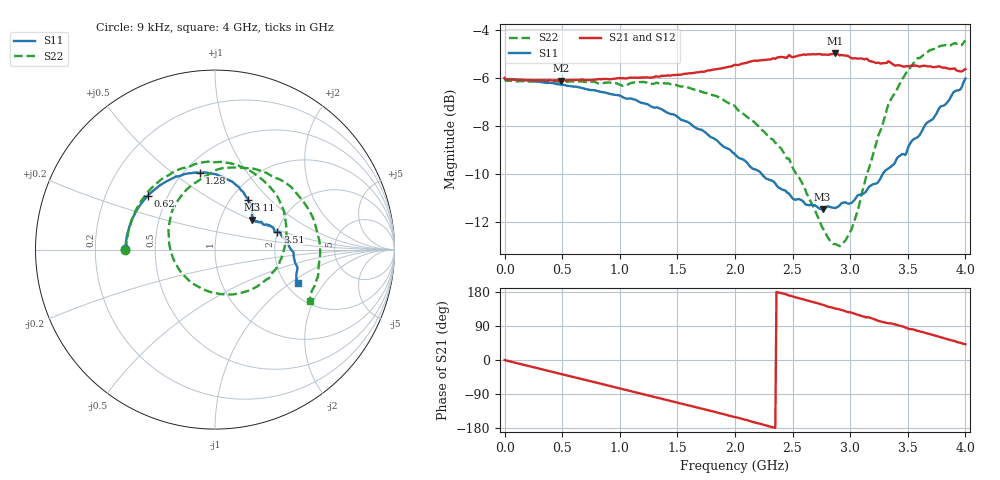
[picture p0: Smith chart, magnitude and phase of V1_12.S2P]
! ZVRE, 3.40
! symbol freq-unit parameter-type data-format keyword impedance-ohm
#  HZ  S  RI  R  50
! freq  reS11  imS11  reS21  imS21  reS12  imS12  reS22  imS22
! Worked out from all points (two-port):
!   401 points, 9 kHz to 4 GHz, reference 50 ohm
!   highest |S21| = -4.96 dB at 2.87 GHz (marker M1); lowest = -6.1 dB at 490 MHz (marker M2)
!   |S21| within 3 dB of the highest: start of sweep to end of sweep
!   lowest |S11| = -11.5 dB at 2.76 GHz (marker M3), VSWR 1.73, Z = 70.9 + j25.5 ohm
!   |S11| at or under -10 dB: 2.232 GHz to 3.283 GHz (1.051 GHz wide, 38.1 % of centre)
!   |S22| runs from -13.0 to -4.4 dB; largest |S21 - S12| = 0.02
!   S11 on the Smith chart (normalised r, x): 9 kHz: 0.33, +0.00; 620 MHz: 0.39, +0.30; 1.28 GHz: 0.59, +0.63; 2.11 GHz: 1.19, +0.75; 3.51 GHz: 2.00, +0.46; 4 GHz: 2.34, -1.15
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9000  -0.4999 0.000718  0.5014 0.000349  0.5019 -0.00206  -0.5 -0.000897
4.900079e8  -0.4173 0.2476  0.3952 -0.2977  0.3997 -0.2964  -0.407 0.2766
6.200076e8  -0.3754 0.3004  0.3407 -0.3608  0.3453 -0.3613  -0.3588 0.3379
6.700075e8  -0.3573 0.3171  0.3165 -0.3831  0.3216 -0.3821  -0.3364 0.3597
9.900068e8  -0.2215 0.4047  0.1363 -0.4818  0.1393 -0.4839  -0.1703 0.4557
1.280006e9  -0.0854 0.4281  -0.0528 -0.4996  -0.0504 -0.5021  0.00449 0.4875
1.340006e9  -0.0557 0.43  -0.0909 -0.4958  -0.0898 -0.5002  0.0431 0.4866
1.660005e9  0.0768 0.3871  -0.291 -0.4244  -0.2899 -0.4269  0.2452 0.4048
2.000004e9  0.1667 0.3048  -0.4648 -0.2626  -0.4651 -0.2641  0.3869 0.2047
2.110004e9  0.1828 0.2783  -0.5047 -0.192  -0.5061 -0.1941  0.3964 0.1219
2.400004e9  0.2075 0.209  -0.5533 0.0317  -0.5545 0.0294  0.342 -0.1036
2.670003e9  0.211 0.1725  -0.5021 0.2507  -0.5077 0.2459  0.1166 -0.2474
2.760003e9  0.2083 0.1669  -0.465 0.3127  -0.4714 0.3097  0.0129 -0.2441
2.870003e9  0.2137 0.1628  -0.4053 0.3934  -0.4125 0.386  -0.1235 -0.1896
2.990002e9  0.2239 0.1587  -0.3263 0.4491  -0.3293 0.4499  -0.2312 -0.0533
3.110002e9  0.2421 0.1552  -0.2332 0.4971  -0.2438 0.495  -0.2544 0.1466
3.200002e9  0.2588 0.1543  -0.1725 0.5128  -0.1795 0.5151  -0.1971 0.2869
3.340001e9  0.2967 0.1343  -0.0636 0.5382  -0.0651 0.541  0.0142 0.4466
3.510001e9  0.3482 0.0997  0.076 0.5253  0.0605 0.5382  0.332 0.4009
3.650001e9  0.3961 0.0542  0.165 0.5048  0.1667 0.5133  0.5039 0.2511
3.760001e9  0.428 -0.00474  0.2463 0.4687  0.2498 0.4754  0.5735 0.0778
4e9  0.4647 -0.1838  0.3913 0.3469  0.3991 0.3411  0.5268 -0.2868
